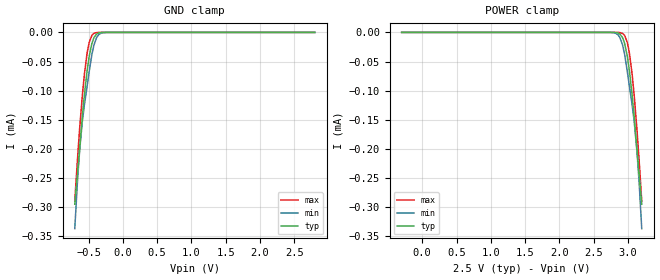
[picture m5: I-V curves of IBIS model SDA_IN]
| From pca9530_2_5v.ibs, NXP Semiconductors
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[Model]   SDA_IN
Model_type Input
Vinh=1.75
Vinl=0.75
C_comp   4p   3.8p   4.2p
[Temperature Range] 27   85   -40
[Voltage Range]   2.5   2.2   2.8
[GND Clamp]
-700mV    -295uA     -337uA     -289.5uA
-660mV    -241.9uA   -254.1uA   -216.6uA
-630mV    -200.9uA   -204uA     -166.8uA
-590mV    -145.3uA   -153.2uA   -108.4uA
-560mV    -107.6uA   -124.5uA   -71.97uA
-520mV    -65.58uA   -92.63uA   -35.3uA
-490mV    -41.22uA   -67.38uA   -17.26uA
-450mV    -18.67uA   -37.44uA   -5.001uA
-420mV    -8.79uA    -21.47uA   -1.619uA
-350mV    -920.5nA   -3.647uA   -77.68nA
-210mV    -3.652nA   -27.14nA   -101.2pA
2.8V      6.71pA     20.63pA    5.609pA
[POWER Clamp]
-300mV    6.71pA     20.63pA    5.609pA
2.71V     -3.652nA   -27.14nA   -101.2pA
2.85V     -920.5nA   -3.647uA   -77.68nA
2.92V     -8.79uA    -21.47uA   -1.619uA
2.95V     -18.67uA   -37.44uA   -5.001uA
2.99V     -41.22uA   -67.38uA   -17.26uA
3.02V     -65.58uA   -92.63uA   -35.3uA
3.06V     -107.6uA   -124.5uA   -71.97uA
3.09V     -145.3uA   -153.2uA   -108.4uA
3.13V     -200.9uA   -204uA     -166.8uA
3.16V     -241.9uA   -254.1uA   -216.6uA
3.2V      -295uA     -337uA     -289.5uA
